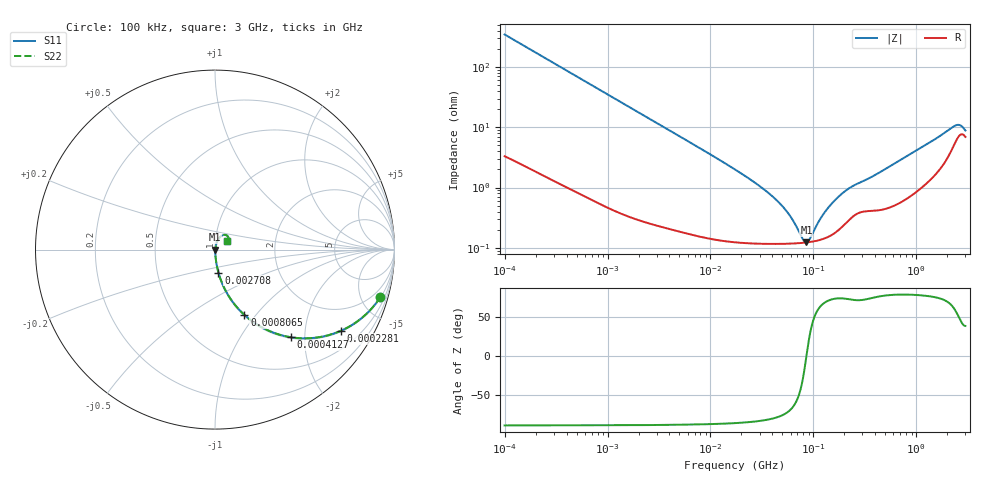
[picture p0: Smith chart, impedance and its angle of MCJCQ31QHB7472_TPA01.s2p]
! MCJCQ31QHB7472_TPA01  S-PARAMETER MODEL  ( Standard Model )
! Model Generated by TAIYO YUDEN Corporation (http://www.ty-top.com)
! Version 1.0
! TAIYO YUDEN Control No. 220601
! Copyright(c) 2015 TAIYO YUDEN CO.,LTD. All Rights Reserved.
! Product Description (link to TY-COMPAS)
! https://ds.yuden.co.jp/TYCOMPAS/or/detail?pn=MCJCQ31QHB7472KTPA01&u=M
! Products Name : Multilayer Ceramic Capacitors
! Characteristics :
!  Capacitance : 4700 [pF] , Rated Voltage : 250 [V] , TCC : X7R
!  Case Size : 3.2 x 1.6 / 0.126 x 0.063 [mm/inch] , Thickness : 1.15 / 0.045 [mm/inch]
!  (Conditions: Temperature = 25 [degC] , DC Bias Voltage = 0 [V])
! External Node Assignments :
!  1  o---| |---o  2
! GND o---------o GND
! Frequency Range : 100kHz  -  3GHz  [ 401 STEP ]
# MHZ S RI R 50
! Freq[MHz].  S11 Real  S11 Imag  S21 Real  S21 Imag  S12 Real  S12 Imag  S22 Real  S22 Imag
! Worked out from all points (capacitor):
!   401 points, 100 kHz to 3 GHz, reference 50 ohm
!   read as one part in series: C = 4.57 nF near 105.3 kHz
!   lowest |Z| = 123 mohm at 85.61 MHz (marker M1)
!   series resonance near 85.7 MHz, so ESL is about 760 pH
!   S11 on the Smith chart (normalised r, x): 100 kHz: 1.07, -6.96; 228.1 kHz: 1.03, -3.07; 412.7 kHz: 1.02, -1.70; 806.5 kHz: 1.01, -0.88; 2.708 MHz: 1.00, -0.26; 3 GHz: 1.14, +0.11
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0.1  0.9216 -0.2641  0.0784 0.2641  0.0784 0.2641  0.9216 -0.2641
0.151038  0.8397 -0.3619  0.1603 0.3619  0.1603 0.3619  0.8397 -0.3619
0.228123  0.6997 -0.4531  0.3003 0.4531  0.3003 0.4531  0.6997 -0.4531
0.412671  0.421 -0.488  0.579 0.488  0.579 0.488  0.421 -0.488
0.562235  0.284 -0.445  0.716 0.445  0.716 0.445  0.284 -0.445
0.806524  0.1638 -0.3638  0.8362 0.3638  0.8362 0.3638  0.1638 -0.3638
1.350433  0.0673 -0.2435  0.9327 0.2435  0.9327 0.2435  0.0673 -0.2435
2.708188  0.0192 -0.1283  0.9808 0.1283  0.9808 0.1283  0.0192 -0.1283
3.161081  0.0147 -0.1105  0.9853 0.1105  0.9853 0.1105  0.0147 -0.1105
17.7727  0.0016 -0.0193  0.9984 0.0193  0.9984 0.0193  0.0016 -0.0193
31.3325  0.00127 -0.00996  0.9987 0.00996  0.9987 0.00996  0.00127 -0.00996
46.11977  0.00119 -0.00556  0.9988 0.00556  0.9988 0.00556  0.00119 -0.00556
58.15973  0.00118 -0.00336  0.9988 0.00336  0.9988 0.00336  0.00118 -0.00336
79.23846  0.00121 -0.000666  0.9988 0.000666  0.9988 0.000666  0.00121 -0.000666
85.60801  0.00123 -9.28e-06  0.9988 9.28e-06  0.9988 9.28e-06  0.00123 -9.28e-06
97.38194  0.00127 0.00109  0.9987 -0.00109  0.9987 -0.00109  0.00127 0.00109
129.3002  0.00145 0.00364  0.9986 -0.00364  0.9986 -0.00364  0.00145 0.00364
185.4806  0.00219 0.00735  0.9978 -0.00735  0.9978 -0.00735  0.00219 0.00735
547.5153  0.00509 0.0216  0.9949 -0.0216  0.9949 -0.0216  0.00509 0.0216
2318.426  0.0549 0.0819  0.9451 -0.0819  0.9451 -0.0819  0.0549 0.0819
2637.286  0.0738 0.0696  0.9262 -0.0696  0.9262 -0.0696  0.0738 0.0696
3000  0.0674 0.0479  0.9326 -0.0479  0.9326 -0.0479  0.0674 0.0479
